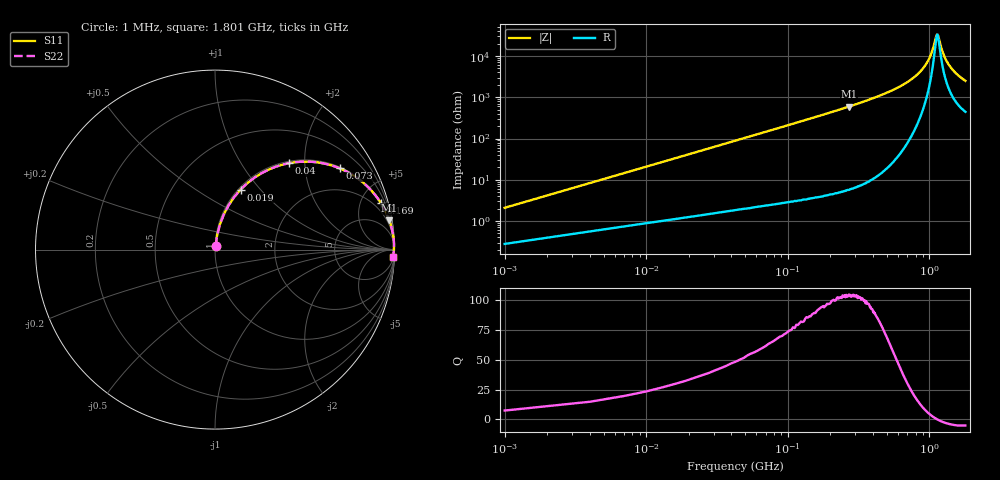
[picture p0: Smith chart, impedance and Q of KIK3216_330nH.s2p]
!version-2
!date-01.2022
!Series
# MHz S RI R 50
!Freq ReS11 ImS11 ReS21 ImS21 ReS12 ImS12 ReS22 ImS22
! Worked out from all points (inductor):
!   601 points, 1 MHz to 1.801 GHz, reference 50 ohm
!   read as one part in series: L = 330 nH near 10 MHz
!   highest Q = 104 at 271 MHz (marker M1), where L = 350 nH
!   self-resonance near 1.141 GHz
!   S11 on the Smith chart (normalised r, x): 1 MHz: 1.01, +0.04; 19 MHz: 1.02, +0.79; 40 MHz: 1.04, +1.66; 73 MHz: 1.05, +3.04; 169 MHz: 1.08, +7.17; 1.801 GHz: 10, -49
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1  0.00322 0.0206  0.9968 -0.0206  0.9968 -0.0206  0.00322 0.0206
13  0.0758 0.2467  0.9242 -0.2467  0.9242 -0.2467  0.0758 0.2467
19  0.1421 0.334  0.8579 -0.334  0.8579 -0.334  0.1421 0.334
28  0.2578 0.4248  0.7422 -0.4248  0.7422 -0.4248  0.2578 0.4248
40  0.4101 0.4813  0.5899 -0.4813  0.5899 -0.4813  0.4101 0.4813
55  0.5654 0.4867  0.4346 -0.4867  0.4346 -0.4867  0.5654 0.4867
73  0.6951 0.4525  0.3049 -0.4525  0.3049 -0.4525  0.6951 0.4525
112  0.8429 0.3574  0.1571 -0.3574  0.1571 -0.3574  0.8429 0.3574
169  0.9254 0.2575  0.0746 -0.2575  0.0746 -0.2575  0.9254 0.2575
271  0.9711 0.1628  0.0289 -0.1628  0.0289 -0.1628  0.9711 0.1628
301  0.9769 0.1454  0.0231 -0.1454  0.0231 -0.1454  0.9769 0.1454
601  0.9954 0.0576  0.00456 -0.0576  0.00456 -0.0576  0.9954 0.0576
778  0.9973 0.033  0.00271 -0.033  0.00271 -0.033  0.9973 0.033
901  0.9976 0.02  0.00241 -0.02  0.00241 -0.02  0.9976 0.02
1021  0.9974 0.00939  0.00255 -0.00939  0.00255 -0.00939  0.9974 0.00939
1132  0.997 0.000722  0.00296 -0.000722  0.00296 -0.000722  0.997 0.000722
1156  0.9969 -0.00103  0.00307 0.00103  0.00307 0.00103  0.9969 -0.00103
1201  0.9967 -0.00422  0.00331 0.00422  0.00331 0.00422  0.9967 -0.00422
1255  0.9964 -0.00789  0.00363 0.00789  0.00363 0.00789  0.9964 -0.00789
1318  0.996 -0.012  0.00404 0.012  0.00404 0.012  0.996 -0.012
1501  0.9945 -0.023  0.00551 0.023  0.00551 0.023  0.9945 -0.023
1801  0.9914 -0.0387  0.00856 0.0387  0.00856 0.0387  0.9914 -0.0387
